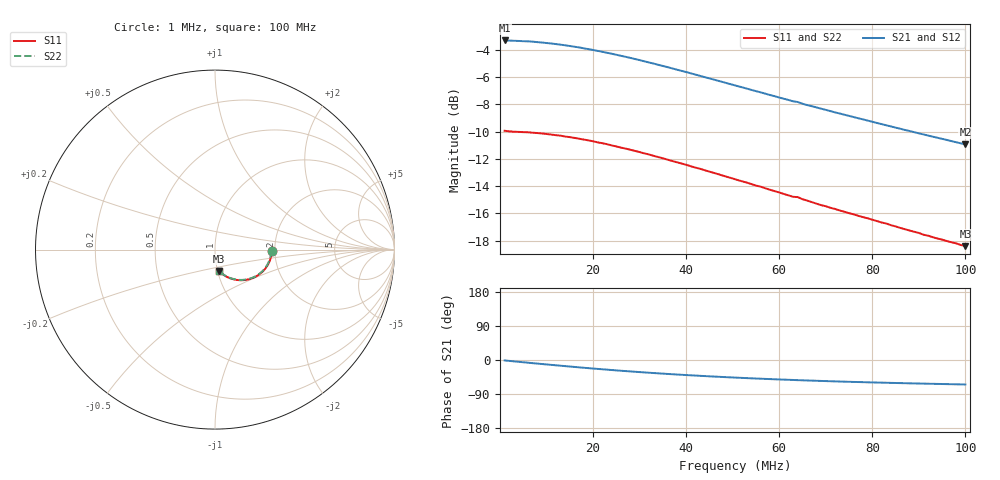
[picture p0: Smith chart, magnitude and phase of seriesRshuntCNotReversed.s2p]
# Hz S RI R 50.0
! written by SimSmith version 18.3b
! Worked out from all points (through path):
!   100 points, 1 MHz to 100 MHz, reference 50 ohm
!   highest |S21| = -3.31 dB at 1 MHz (marker M1); lowest = -10.9 dB at 100 MHz (marker M2)
!   group delay of S21, straight-line fit = 1.72 ns
!   lowest |S11| = -18.4 dB at 100 MHz (marker M3), VSWR 1.27, Z = 50.6 - j12.2 ohm
!   |S11| at or under -10 dB: 2.749 MHz to end of sweep
!   |S22| runs from -18.5 to -10.0 dB; largest |S21 - S12| = 0
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1000000  0.3184 -0.00791  0.6833 -0.0144  0.6833 -0.0144  0.3152 -0.00785
2000000  0.3167 -0.0135  0.6821 -0.0281  0.6821 -0.0281  0.3134 -0.013
6000000  0.3116 -0.043  0.6733 -0.0837  0.6733 -0.0837  0.3088 -0.0422
9000000  0.3049 -0.0634  0.6603 -0.123  0.6603 -0.123  0.3021 -0.0623
1.3e7  0.2926 -0.0882  0.637 -0.1714  0.637 -0.1714  0.2903 -0.0869
1.8e7  0.2724 -0.1151  0.5992 -0.2235  0.5992 -0.2235  0.2704 -0.1135
2.2e7  0.2546 -0.1319  0.5651 -0.2576  0.5651 -0.2576  0.2529 -0.1303
2.6e7  0.2348 -0.1456  0.5283 -0.285  0.5283 -0.285  0.2335 -0.1439
3e7  0.2155 -0.1561  0.4916 -0.3059  0.4916 -0.3059  0.2142 -0.1543
3.4e7  0.1961 -0.1631  0.4548 -0.3204  0.4548 -0.3204  0.1951 -0.1614
3.7e7  0.1821 -0.1665  0.4281 -0.3288  0.4281 -0.3288  0.1813 -0.1648
4.2e7  0.1599 -0.1698  0.3861 -0.3365  0.3861 -0.3365  0.1593 -0.1682
4.6e7  0.1434 -0.1707  0.3548 -0.3391  0.3548 -0.3391  0.1428 -0.169
5.1e7  0.1245 -0.1693  0.319 -0.3382  0.319 -0.3382  0.1241 -0.1677
6e7  0.0953 -0.1633  0.2636 -0.3295  0.2636 -0.3295  0.0952 -0.1617
6.3e7  0.0869 -0.1602  0.2476 -0.325  0.2476 -0.325  0.0868 -0.1587
6.4e7  0.0855 -0.1604  0.2432 -0.3255  0.2432 -0.3255  0.0855 -0.1589
6.7e7  0.0764 -0.1566  0.2281 -0.319  0.2281 -0.319  0.0765 -0.1551
7.5e7  0.0586 -0.1475  0.194 -0.3047  0.194 -0.3047  0.0588 -0.1461
8.4e7  0.0426 -0.137  0.1633 -0.2873  0.1633 -0.2873  0.0429 -0.1357
9.2e7  0.0307 -0.1276  0.1406 -0.2715  0.1406 -0.2715  0.0312 -0.1264
1e8  0.0203 -0.1184  0.1218 -0.2568  0.1218 -0.2568  0.0208 -0.1173
